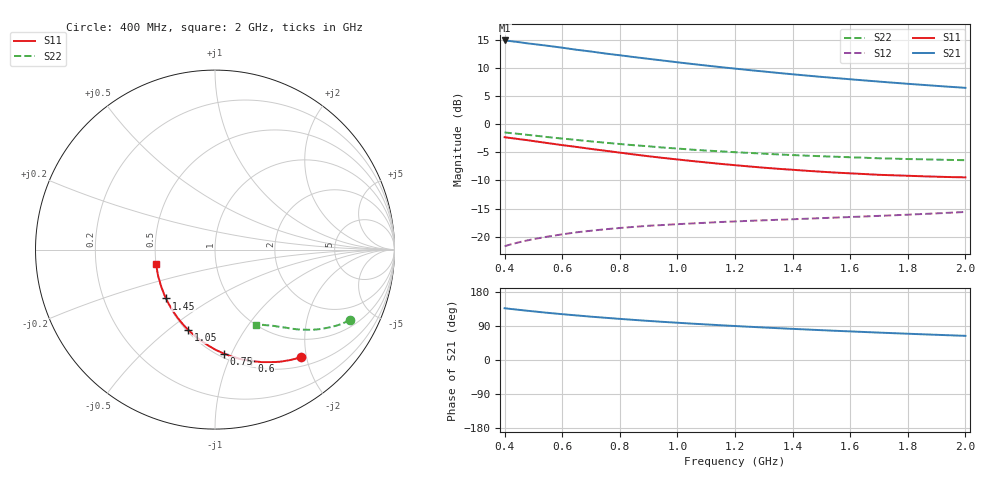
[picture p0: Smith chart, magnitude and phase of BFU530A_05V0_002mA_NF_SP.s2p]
! Filename:  P:\Prog\Test\Noise\ATS_data\Testdata_Net\06 Compressed Noise after Statistics\BFU530A_APG2013_33_A05_05p0V_002mA_SP_CM01_D.sf
! Date/Time: Tue 16/Apr/2013 15:10:59
! BFU530A_APG2013_33_A05_05p0V_1to25mA_NF_CM01_Bias2_R.sf
! Noise Parameter Data File
! BFU530A_APG2013_33_A05_05p0V_1to25mA_NF_CM01
! Date/time: Fri Apr 12 15:27:54 2013
! VAR V_out= 5.001000
! VAR I_out= 2.000000
! VAR V_in= 0.799900
! VAR I_in= 0.020805
! Device data file deembeded for feedlines and parallel
! Original file: \06 Compressed Noise after Statistics\BFU530A_APG2013_33_A05_05p0V_002mA_SP_CM01_R.sf
! Feed-files: PR017V01_150413_Feed1.s2p, PR017V01_150413_Feed2.s2p
! Parallel-file: PR017V01_150413_Par.s2p
# MHz S MA R 50
!  Freq-MHz  S11-mag  S11-arg  S21-mag  S21-arg  S12-mag  S12-arg  S22-mag  S22-arg
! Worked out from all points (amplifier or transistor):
!   37 points, 400 MHz to 2 GHz, reference 50 ohm
!   highest |S21| = 14.9 dB at 400 MHz (marker M1)
!   |S21| within 3 dB of that: start of sweep to 855.9 MHz
!   unconditionally stable (mu >= 1): nowhere
!   at 500 MHz: K = 0.34, MSG = 17.4 dB, |S12| = -20.4 dB
!   at 1.1 GHz: K = 0.68, MSG = 14.0 dB, |S12| = -17.5 dB
!   at 2 GHz: K = 1.00, MSG = 11.1 dB, |S12| = -15.6 dB
!   lowest NFmin = 0.49 dB at 400 MHz
!   S11 on the Smith chart (normalised r, x): 400 MHz: 0.65, -1.91; 600 MHz: 0.56, -1.22; 750 MHz: 0.53, -0.94; 1.05 GHz: 0.51, -0.59; 1.45 GHz: 0.50, -0.32; 2 GHz: 0.50, -0.09
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400  0.7682 -51.3  5.589 136.6  0.08216 61.6  0.8471 -27.6
420  0.7559 -53.5  5.516 134.8  0.08502 60.6  0.8365 -28.6
440  0.7447 -55.7  5.436 133.1  0.08768 59.6  0.8265 -29.6
500  0.7096 -62.0  5.194 128.3  0.09495 57.0  0.7958 -32.2
550  0.6807 -67.2  5.009 124.5  0.1 55.0  0.7698 -34.3
600  0.6531 -71.9  4.818 120.9  0.1047 53.4  0.7468 -36.1
650  0.6291 -76.4  4.618 117.6  0.1092 51.9  0.7263 -37.7
700  0.6039 -81.0  4.454 114.4  0.1128 50.6  0.7049 -39.3
750  0.5816 -85.1  4.274 111.4  0.1163 49.5  0.686 -40.6
850  0.5389 -93.4  3.973 105.8  0.1221 47.7  0.6512 -43.1
900  0.5196 -97.4  3.833 103.1  0.1249 46.9  0.6374 -44.2
950  0.5024 -101.2  3.701 100.7  0.1268 46.4  0.6211 -45.3
1050  0.4714 -108.4  3.452 96.0  0.1309 45.6  0.5952 -47.2
1100  0.4578 -112.0  3.34 93.8  0.1328 45.4  0.584 -48.0
1200  0.4326 -118.9  3.137 89.7  0.1364 45.0  0.5645 -49.7
1300  0.4111 -125.4  2.956 85.8  0.1397 45.0  0.5479 -51.4
1450  0.3855 -135.1  2.719 80.4  0.1444 45.5  0.5258 -53.6
1500  0.3784 -138.2  2.647 78.7  0.146 45.7  0.5197 -54.3
1650  0.3607 -147.2  2.461 73.9  0.1511 46.8  0.5041 -56.6
1750  0.3517 -153.0  2.349 70.8  0.1548 47.6  0.4948 -58.0
1850  0.3446 -158.5  2.249 67.9  0.1589 48.5  0.4883 -59.5
2000  0.3371 -166.7  2.114 63.7  0.1657 49.9  0.4793 -61.8
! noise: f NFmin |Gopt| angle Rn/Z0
400  0.4883  0.508  23.68  0.2011
460  0.5108  0.5102  26.84  0.1938
600  0.5967  0.4511  30.76  0.2086
800  0.5868  0.4539  50.55  0.1611
1000  0.6317  0.4409  64.3  0.1476
1200  0.7035  0.4231  76.7  0.1394
1400  0.753  0.4086  93.98  0.1163
1600  0.8866  0.3972  107.3  0.086
1800  0.7504  0.3665  128.1  0.0778
2000  0.8688  0.3386  137.5  0.0736
